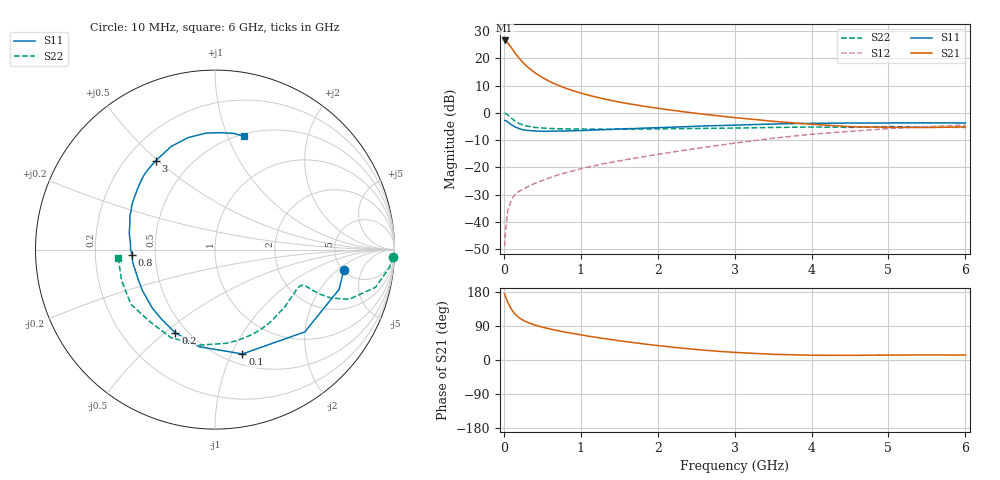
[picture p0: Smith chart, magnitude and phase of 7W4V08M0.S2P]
! Infineon Technologies  Discrete & RF Semiconductors
! BFS17W
! Si NPN RF Bipolar Junction Transistor in SOT323
! VCE = 4 V  IC = 8 mA
! Common Emitter S-Parameters:  August  1999
# GHz  S  MA  R  50
!  f  S11  S21  S12  S22
! GHz  MAG  ANG  MAG  ANG  MAG  ANG  MAG  ANG
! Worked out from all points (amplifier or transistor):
!   36 points, 10 MHz to 6 GHz, reference 50 ohm
!   highest |S21| = 26.5 dB at 10 MHz (marker M1)
!   |S21| within 3 dB of that: start of sweep to 106.1 MHz
!   unconditionally stable (mu >= 1): 455.2 MHz to 2.481 GHz; 4.752 GHz to end of sweep
!   at 250 MHz: K = 0.74, MSG = 23.3 dB, |S12| = -28.1 dB
!   at 1.4 GHz: K = 1.21, MAG = 8.6 dB, |S12| = -18.1 dB
!   at 6 GHz: K = 1.07, MAG = -1.9 dB, |S12| = -4.5 dB
!   S11 on the Smith chart (normalised r, x): 10 MHz: 5.14, -2.43; 100 MHz: 0.60, -1.10; 200 MHz: 0.43, -0.54; 800 MHz: 0.37, -0.03; 3 GHz: 0.32, +0.49; 6 GHz: 0.52, +1.15
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0.01  0.727 -8.8  21.2 174.6  0.0036 83.0  0.9909 -2.4
0.02  0.726 -17.8  20.94 168.5  0.0063 82.7  0.9773 -5.8
0.05  0.6786 -42.5  19.26 152.7  0.016 70.1  0.9188 -13.2
0.1  0.601 -75.3  15.43 133.3  0.0262 59.6  0.7959 -20.4
0.15  0.5482 -99.3  12.26 120.1  0.0324 53.8  0.6976 -22.7
0.2  0.5136 -115.4  9.978 111.4  0.0368 53.2  0.6368 -23.0
0.25  0.4892 -127.3  8.302 105.0  0.0392 52.0  0.5955 -22.7
0.3  0.4779 -136.8  7.093 100.1  0.0436 52.7  0.5714 -22.3
0.4  0.4645 -150.3  5.469 92.4  0.0507 55.3  0.5409 -21.9
0.5  0.4591 -159.1  4.438 86.7  0.0575 57.8  0.5267 -22.1
0.6  0.4591 -166.0  3.723 81.8  0.0645 59.5  0.5169 -22.9
0.8  0.4631 -176.4  2.844 73.5  0.0794 62.3  0.5067 -25.7
0.9  0.4712 179.5  2.54 69.9  0.0862 63.4  0.5038 -27.4
1.1  0.4793 172.0  2.107 62.8  0.102 64.7  0.5025 -31.5
1.3  0.4916 165.5  1.804 56.7  0.1169 65.7  0.4998 -36.1
1.6  0.5121 157.4  1.485 48.1  0.1394 66.8  0.5015 -43.3
2.2  0.5465 142.6  1.109 33.7  0.1917 68.4  0.5125 -59.9
3  0.595 123.7  0.818 20.1  0.2786 66.1  0.5256 -83.4
3.5  0.6245 113.1  0.7 15.0  0.3421 62.2  0.5394 -99.3
4.5  0.6509 94.4  0.558 12.3  0.4579 50.0  0.5411 -132.4
5.5  0.6558 80.7  0.538 13.4  0.5581 37.3  0.5485 -161.8
6  0.6516 75.5  0.552 13.0  0.5971 31.0  0.5406 -174.8
